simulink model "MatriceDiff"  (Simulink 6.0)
settings: Solver=ode45  StartTime=0  StopTime=17*t0  RelTol=1e-3
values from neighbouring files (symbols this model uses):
  b = S/Sm    (= 0.1)    [Constantes.m]    (also in ConstantesBck.m)
  beta = 0.95    [Constantes.m]    (also in ConstantesBck.m; ResCourV1.m = 1; ResCrV1.m = 1; ResEnerV1.m = 1)
  C = 1    [Constantes.m]    (also in ConstantesBck.m)
  gk = 36    [Constantes.m]    (also in ConstantesBck.m; sim_hh.m)
  gl = 0.3    [Constantes.m]    (also in ConstantesBck.m; sim_hh.m)
  gna = 120    [Constantes.m]    (also in ConstantesBck.m; sim_hh.m)
  h0 = 0.5961    [Constantes.m]    (also in ConstantesBck.m)
  m0 = 0.0529    [Constantes.m]    (also in ConstantesBck.m)
  mK = 0    [Constantes.m]    (also in ConstantesBck.m)
  mL = 0    [Constantes.m]    (also in ConstantesBck.m)
  mNa = 0    [Constantes.m]    (also in ConstantesBck.m)
  N = [6,8,5,5,7,1,2,6,9,1,1,9,4,8,8,7]    [Constantes.m]    (also in ConstantesBck.m; ImpedanceZtissus.m = 100; Ztissus.m = 100; charge.m = N(:,2))
  n0 = 0.3177    [Constantes.m]    (also in ConstantesBck.m)
  rapportIE = 10    [Constantes.m]
  Sm = 3.14e-2    (= 0.0314)    [Constantes.m]    (also in ConstantesBck.m = 0.000314)
  t0 = 2E-3    (= 0.002)    [Constantes.m]    (also in ConstantesBck.m = 0.001)
  Vk = -82    [Constantes.m]    (also in ConstantesBck.m)
  Vl = -59    [Constantes.m]    (also in ConstantesBck.m)
  Vna = 45    [Constantes.m]    (also in ConstantesBck.m)
  Vr = -70    [Constantes.m]    (also in ConstantesBck.m)
undefined symbols (not defined in the file or in its folder): ln
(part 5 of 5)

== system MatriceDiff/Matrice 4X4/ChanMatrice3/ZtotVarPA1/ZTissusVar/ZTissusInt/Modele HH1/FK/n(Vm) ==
  note: V
  note: alpha_*(1-n)
  note: beta_n*n
  note: n
  note: n
  Vm : Inport  Port=1  LatchInput=off
  (1-n) : Fcn  Expr=1-u
  Integrator1 : Integrator  InitialCondition=n0
  Product : Product
  Product1 : Product
  Sum1 : Sum  Inputs=+-
  V : Fcn  Expr=u-Vr
  alpha_n : Fcn  Expr=(0.01*(10-u))/(exp((10-u)/10)-1)
  beta_n : Fcn  Expr=0.125*exp(-u/80)
  n : Outport  InitialOutput=0
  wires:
  V/1 -> alpha_n/1, beta_n/1
  alpha_n/1 -> Product/2
  (1-n)/1 -> Product/1
  beta_n/1 -> Product1/1
  Product/1 -> Sum1/1
  Product1/1 -> Sum1/2
  Sum1/1 -> Integrator1/1
  Integrator1/1 -> (1-n)/1, Product1/2, n/1
  Vm/1 -> V/1

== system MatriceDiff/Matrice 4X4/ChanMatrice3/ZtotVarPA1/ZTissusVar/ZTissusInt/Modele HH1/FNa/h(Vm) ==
  note: h
  note: h
  note: beta_h*h
  note: alpha_h*(1-h)
  note: V
  Vm : Inport  Port=1  LatchInput=off
  (1-h) : Fcn  Expr=1-u
  Integrator1 : Integrator  InitialCondition=h0
  Product : Product
  Product1 : Product
  Sum1 : Sum  Inputs=+-
  V : Fcn  Expr=u-Vr
  alpha_h : Fcn  Expr=0.07*exp(-u/20)
  beta_h : Fcn  Expr=1/(exp((30-u)/10)+1)
  h : Outport  InitialOutput=0
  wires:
  Vm/1 -> V/1
  Integrator1/1 -> h/1, Product1/2, (1-h)/1
  Sum1/1 -> Integrator1/1
  Product1/1 -> Sum1/2
  Product/1 -> Sum1/1
  beta_h/1 -> Product1/1
  (1-h)/1 -> Product/1
  alpha_h/1 -> Product/2
  V/1 -> beta_h/1, alpha_h/1

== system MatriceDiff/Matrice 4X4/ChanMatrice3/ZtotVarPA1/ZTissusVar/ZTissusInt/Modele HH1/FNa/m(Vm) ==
  note: m
  note: m
  note: beta_m*m
  note: alpha_m*(1-m)
  note: V
  Vm : Inport  Port=1  LatchInput=off
  (1-m) : Fcn  Expr=1-u
  Integrator1 : Integrator  InitialCondition=m0
  Product : Product
  Product1 : Product
  Sum1 : Sum  Inputs=+-
  V : Fcn  Expr=u-Vr
  alpha_m : Fcn  Expr=(0.1*(25-u))/(exp((25-u)/10)-1)
  beta_m : Fcn  Expr=4*exp(-u/18)
  n : Outport  InitialOutput=0
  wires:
  Vm/1 -> V/1
  Integrator1/1 -> n/1, Product1/2, (1-m)/1
  Sum1/1 -> Integrator1/1
  Product1/1 -> Sum1/2
  Product/1 -> Sum1/1
  beta_m/1 -> Product1/1
  (1-m)/1 -> Product/1
  alpha_m/1 -> Product/2
  V/1 -> beta_m/1, alpha_m/1

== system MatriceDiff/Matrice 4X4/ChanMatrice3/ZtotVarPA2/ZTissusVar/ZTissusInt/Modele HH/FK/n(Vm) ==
  note: V
  note: alpha_*(1-n)
  note: beta_n*n
  note: n
  note: n
  Vm : Inport  Port=1  LatchInput=off
  (1-n) : Fcn  Expr=1-u
  Integrator1 : Integrator  InitialCondition=n0
  Product : Product
  Product1 : Product
  Sum1 : Sum  Inputs=+-
  V : Fcn  Expr=u-Vr
  alpha_n : Fcn  Expr=(0.01*(10-u))/(exp((10-u)/10)-1)
  beta_n : Fcn  Expr=0.125*exp(-u/80)
  n : Outport  InitialOutput=0
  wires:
  V/1 -> alpha_n/1, beta_n/1
  alpha_n/1 -> Product/2
  (1-n)/1 -> Product/1
  beta_n/1 -> Product1/1
  Product/1 -> Sum1/1
  Product1/1 -> Sum1/2
  Sum1/1 -> Integrator1/1
  Integrator1/1 -> (1-n)/1, Product1/2, n/1
  Vm/1 -> V/1

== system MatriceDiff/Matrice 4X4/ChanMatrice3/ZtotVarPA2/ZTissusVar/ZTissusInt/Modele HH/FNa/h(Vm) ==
  note: h
  note: h
  note: beta_h*h
  note: alpha_h*(1-h)
  note: V
  Vm : Inport  Port=1  LatchInput=off
  (1-h) : Fcn  Expr=1-u
  Integrator1 : Integrator  InitialCondition=h0
  Product : Product
  Product1 : Product
  Sum1 : Sum  Inputs=+-
  V : Fcn  Expr=u-Vr
  alpha_h : Fcn  Expr=0.07*exp(-u/20)
  beta_h : Fcn  Expr=1/(exp((30-u)/10)+1)
  h : Outport  InitialOutput=0
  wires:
  Vm/1 -> V/1
  Integrator1/1 -> h/1, Product1/2, (1-h)/1
  Sum1/1 -> Integrator1/1
  Product1/1 -> Sum1/2
  Product/1 -> Sum1/1
  beta_h/1 -> Product1/1
  (1-h)/1 -> Product/1
  alpha_h/1 -> Product/2
  V/1 -> beta_h/1, alpha_h/1

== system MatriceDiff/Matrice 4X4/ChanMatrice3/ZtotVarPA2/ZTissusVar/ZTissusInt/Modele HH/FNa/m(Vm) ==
  note: m
  note: m
  note: beta_m*m
  note: alpha_m*(1-m)
  note: V
  Vm : Inport  Port=1  LatchInput=off
  (1-m) : Fcn  Expr=1-u
  Integrator1 : Integrator  InitialCondition=m0
  Product : Product
  Product1 : Product
  Sum1 : Sum  Inputs=+-
  V : Fcn  Expr=u-Vr
  alpha_m : Fcn  Expr=(0.1*(25-u))/(exp((25-u)/10)-1)
  beta_m : Fcn  Expr=4*exp(-u/18)
  n : Outport  InitialOutput=0
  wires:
  Vm/1 -> V/1
  Integrator1/1 -> n/1, Product1/2, (1-m)/1
  Sum1/1 -> Integrator1/1
  Product1/1 -> Sum1/2
  Product/1 -> Sum1/1
  beta_m/1 -> Product1/1
  (1-m)/1 -> Product/1
  alpha_m/1 -> Product/2
  V/1 -> beta_m/1, alpha_m/1

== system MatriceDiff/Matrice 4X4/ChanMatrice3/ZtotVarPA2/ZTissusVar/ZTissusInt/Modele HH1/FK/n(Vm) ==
  note: V
  note: alpha_*(1-n)
  note: beta_n*n
  note: n
  note: n
  Vm : Inport  Port=1  LatchInput=off
  (1-n) : Fcn  Expr=1-u
  Integrator1 : Integrator  InitialCondition=n0
  Product : Product
  Product1 : Product
  Sum1 : Sum  Inputs=+-
  V : Fcn  Expr=u-Vr
  alpha_n : Fcn  Expr=(0.01*(10-u))/(exp((10-u)/10)-1)
  beta_n : Fcn  Expr=0.125*exp(-u/80)
  n : Outport  InitialOutput=0
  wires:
  V/1 -> alpha_n/1, beta_n/1
  alpha_n/1 -> Product/2
  (1-n)/1 -> Product/1
  beta_n/1 -> Product1/1
  Product/1 -> Sum1/1
  Product1/1 -> Sum1/2
  Sum1/1 -> Integrator1/1
  Integrator1/1 -> (1-n)/1, Product1/2, n/1
  Vm/1 -> V/1

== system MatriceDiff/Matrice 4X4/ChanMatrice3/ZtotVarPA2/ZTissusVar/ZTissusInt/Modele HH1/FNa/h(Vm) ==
  note: h
  note: h
  note: beta_h*h
  note: alpha_h*(1-h)
  note: V
  Vm : Inport  Port=1  LatchInput=off
  (1-h) : Fcn  Expr=1-u
  Integrator1 : Integrator  InitialCondition=h0
  Product : Product
  Product1 : Product
  Sum1 : Sum  Inputs=+-
  V : Fcn  Expr=u-Vr
  alpha_h : Fcn  Expr=0.07*exp(-u/20)
  beta_h : Fcn  Expr=1/(exp((30-u)/10)+1)
  h : Outport  InitialOutput=0
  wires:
  Vm/1 -> V/1
  Integrator1/1 -> h/1, Product1/2, (1-h)/1
  Sum1/1 -> Integrator1/1
  Product1/1 -> Sum1/2
  Product/1 -> Sum1/1
  beta_h/1 -> Product1/1
  (1-h)/1 -> Product/1
  alpha_h/1 -> Product/2
  V/1 -> beta_h/1, alpha_h/1

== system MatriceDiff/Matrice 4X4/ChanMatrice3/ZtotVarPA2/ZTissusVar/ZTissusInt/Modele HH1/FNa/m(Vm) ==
  note: m
  note: m
  note: beta_m*m
  note: alpha_m*(1-m)
  note: V
  Vm : Inport  Port=1  LatchInput=off
  (1-m) : Fcn  Expr=1-u
  Integrator1 : Integrator  InitialCondition=m0
  Product : Product
  Product1 : Product
  Sum1 : Sum  Inputs=+-
  V : Fcn  Expr=u-Vr
  alpha_m : Fcn  Expr=(0.1*(25-u))/(exp((25-u)/10)-1)
  beta_m : Fcn  Expr=4*exp(-u/18)
  n : Outport  InitialOutput=0
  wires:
  Vm/1 -> V/1
  Integrator1/1 -> n/1, Product1/2, (1-m)/1
  Sum1/1 -> Integrator1/1
  Product1/1 -> Sum1/2
  Product/1 -> Sum1/1
  beta_m/1 -> Product1/1
  (1-m)/1 -> Product/1
  alpha_m/1 -> Product/2
  V/1 -> beta_m/1, alpha_m/1

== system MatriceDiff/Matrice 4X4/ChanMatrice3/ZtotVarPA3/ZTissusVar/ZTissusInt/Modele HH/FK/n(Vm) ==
  note: V
  note: alpha_*(1-n)
  note: beta_n*n
  note: n
  note: n
  Vm : Inport  Port=1  LatchInput=off
  (1-n) : Fcn  Expr=1-u
  Integrator1 : Integrator  InitialCondition=n0
  Product : Product
  Product1 : Product
  Sum1 : Sum  Inputs=+-
  V : Fcn  Expr=u-Vr
  alpha_n : Fcn  Expr=(0.01*(10-u))/(exp((10-u)/10)-1)
  beta_n : Fcn  Expr=0.125*exp(-u/80)
  n : Outport  InitialOutput=0
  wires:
  V/1 -> alpha_n/1, beta_n/1
  alpha_n/1 -> Product/2
  (1-n)/1 -> Product/1
  beta_n/1 -> Product1/1
  Product/1 -> Sum1/1
  Product1/1 -> Sum1/2
  Sum1/1 -> Integrator1/1
  Integrator1/1 -> (1-n)/1, Product1/2, n/1
  Vm/1 -> V/1

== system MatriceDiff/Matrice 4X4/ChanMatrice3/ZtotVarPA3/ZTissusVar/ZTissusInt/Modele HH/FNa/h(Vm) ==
  note: h
  note: h
  note: beta_h*h
  note: alpha_h*(1-h)
  note: V
  Vm : Inport  Port=1  LatchInput=off
  (1-h) : Fcn  Expr=1-u
  Integrator1 : Integrator  InitialCondition=h0
  Product : Product
  Product1 : Product
  Sum1 : Sum  Inputs=+-
  V : Fcn  Expr=u-Vr
  alpha_h : Fcn  Expr=0.07*exp(-u/20)
  beta_h : Fcn  Expr=1/(exp((30-u)/10)+1)
  h : Outport  InitialOutput=0
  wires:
  Vm/1 -> V/1
  Integrator1/1 -> h/1, Product1/2, (1-h)/1
  Sum1/1 -> Integrator1/1
  Product1/1 -> Sum1/2
  Product/1 -> Sum1/1
  beta_h/1 -> Product1/1
  (1-h)/1 -> Product/1
  alpha_h/1 -> Product/2
  V/1 -> beta_h/1, alpha_h/1

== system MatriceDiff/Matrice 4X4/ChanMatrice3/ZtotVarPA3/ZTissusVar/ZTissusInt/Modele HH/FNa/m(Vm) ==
  note: m
  note: m
  note: beta_m*m
  note: alpha_m*(1-m)
  note: V
  Vm : Inport  Port=1  LatchInput=off
  (1-m) : Fcn  Expr=1-u
  Integrator1 : Integrator  InitialCondition=m0
  Product : Product
  Product1 : Product
  Sum1 : Sum  Inputs=+-
  V : Fcn  Expr=u-Vr
  alpha_m : Fcn  Expr=(0.1*(25-u))/(exp((25-u)/10)-1)
  beta_m : Fcn  Expr=4*exp(-u/18)
  n : Outport  InitialOutput=0
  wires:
  Vm/1 -> V/1
  Integrator1/1 -> n/1, Product1/2, (1-m)/1
  Sum1/1 -> Integrator1/1
  Product1/1 -> Sum1/2
  Product/1 -> Sum1/1
  beta_m/1 -> Product1/1
  (1-m)/1 -> Product/1
  alpha_m/1 -> Product/2
  V/1 -> beta_m/1, alpha_m/1

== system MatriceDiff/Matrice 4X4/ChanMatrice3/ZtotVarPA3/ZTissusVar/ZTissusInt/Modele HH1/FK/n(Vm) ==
  note: V
  note: alpha_*(1-n)
  note: beta_n*n
  note: n
  note: n
  Vm : Inport  Port=1  LatchInput=off
  (1-n) : Fcn  Expr=1-u
  Integrator1 : Integrator  InitialCondition=n0
  Product : Product
  Product1 : Product
  Sum1 : Sum  Inputs=+-
  V : Fcn  Expr=u-Vr
  alpha_n : Fcn  Expr=(0.01*(10-u))/(exp((10-u)/10)-1)
  beta_n : Fcn  Expr=0.125*exp(-u/80)
  n : Outport  InitialOutput=0
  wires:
  V/1 -> alpha_n/1, beta_n/1
  alpha_n/1 -> Product/2
  (1-n)/1 -> Product/1
  beta_n/1 -> Product1/1
  Product/1 -> Sum1/1
  Product1/1 -> Sum1/2
  Sum1/1 -> Integrator1/1
  Integrator1/1 -> (1-n)/1, Product1/2, n/1
  Vm/1 -> V/1

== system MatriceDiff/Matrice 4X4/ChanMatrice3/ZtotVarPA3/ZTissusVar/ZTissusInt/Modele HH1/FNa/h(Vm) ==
  note: h
  note: h
  note: beta_h*h
  note: alpha_h*(1-h)
  note: V
  Vm : Inport  Port=1  LatchInput=off
  (1-h) : Fcn  Expr=1-u
  Integrator1 : Integrator  InitialCondition=h0
  Product : Product
  Product1 : Product
  Sum1 : Sum  Inputs=+-
  V : Fcn  Expr=u-Vr
  alpha_h : Fcn  Expr=0.07*exp(-u/20)
  beta_h : Fcn  Expr=1/(exp((30-u)/10)+1)
  h : Outport  InitialOutput=0
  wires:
  Vm/1 -> V/1
  Integrator1/1 -> h/1, Product1/2, (1-h)/1
  Sum1/1 -> Integrator1/1
  Product1/1 -> Sum1/2
  Product/1 -> Sum1/1
  beta_h/1 -> Product1/1
  (1-h)/1 -> Product/1
  alpha_h/1 -> Product/2
  V/1 -> beta_h/1, alpha_h/1

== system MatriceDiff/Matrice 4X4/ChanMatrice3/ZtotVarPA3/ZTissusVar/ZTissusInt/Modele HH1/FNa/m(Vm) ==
  note: m
  note: m
  note: beta_m*m
  note: alpha_m*(1-m)
  note: V
  Vm : Inport  Port=1  LatchInput=off
  (1-m) : Fcn  Expr=1-u
  Integrator1 : Integrator  InitialCondition=m0
  Product : Product
  Product1 : Product
  Sum1 : Sum  Inputs=+-
  V : Fcn  Expr=u-Vr
  alpha_m : Fcn  Expr=(0.1*(25-u))/(exp((25-u)/10)-1)
  beta_m : Fcn  Expr=4*exp(-u/18)
  n : Outport  InitialOutput=0
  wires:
  Vm/1 -> V/1
  Integrator1/1 -> n/1, Product1/2, (1-m)/1
  Sum1/1 -> Integrator1/1
  Product1/1 -> Sum1/2
  Product/1 -> Sum1/1
  beta_m/1 -> Product1/1
  (1-m)/1 -> Product/1
  alpha_m/1 -> Product/2
  V/1 -> beta_m/1, alpha_m/1

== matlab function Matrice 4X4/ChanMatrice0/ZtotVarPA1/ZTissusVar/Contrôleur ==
function [y,temp] = fcn(u,calc)
% This block supports an embeddable subset of the MATLAB language.
% See the help menu for details. 

if u == 0
    y = 0;
    temp = 1E-6;
else
    y = calc;
    temp = u;
end

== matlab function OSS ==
function [S0,Ref0,S1,Ref1,S2,Ref2,S3,Ref3,S4,Ref4,S5,Ref5,S6,Ref6,S7,Ref7,S8,Ref8,S9,Ref9,S10,Ref10,S11,Ref11,S12,Ref12,S13,Ref13,S14,Ref14,S15,Ref15,MatCourant] = fcn(u0,u1,u2,u3,u4,u5,u6,u7,u8,u9,u10,u11,u12,u13,u14,u15,tc0,tc1,tc2,dyn,rst)
%Fonction qui détermine les endroits à stimuler pour obtenir une puissance 
%moyenne par canal minimal

%Valeur utilisée
Vdd=3.3*3.14e-2*(1-0.1)*1000; %mV
Imax=200E-6;

%Enregistrement de l'indice et de l'amplitude pour chaque canal
IndAmpChan0=[1,2,3,4;u0,u1,u2,u3];
IndAmpChan1=[5,6,7,8;u4,u5,u6,u7];
IndAmpChan2=[9,10,11,12;u8,u9,u10,u11];
IndAmpChan3=[13,14,15,16;u12,u13,u14,u15];

%Premier tri
for k=1:2
    for i=1:3
        if(IndAmpChan0(2,i)>IndAmpChan0(2,i+1))
            temp=IndAmpChan0(:,i+1);
            IndAmpChan0(:,i+1)=IndAmpChan0(:,i);
            IndAmpChan0(:,i)=temp;        
        end
        if(IndAmpChan1(2,i)<IndAmpChan1(2,i+1))
            temp=IndAmpChan1(:,i+1);
            IndAmpChan1(:,i+1)=IndAmpChan1(:,i);
            IndAmpChan1(:,i)=temp;        
        end    
        if(IndAmpChan2(2,i)>IndAmpChan2(2,i+1))
            temp=IndAmpChan2(:,i+1);
            IndAmpChan2(:,i+1)=IndAmpChan2(:,i);
            IndAmpChan2(:,i)=temp;        
        end    
        if(IndAmpChan3(2,i)<IndAmpChan3(2,i+1))
            temp=IndAmpChan3(:,i+1);
            IndAmpChan3(:,i+1)=IndAmpChan3(:,i);
            IndAmpChan3(:,i)=temp;        
        end        
    end
end

%On regroupe les lignes 2 par deux
sump1=[0,0,0,0];
sump2=[0,0,0,0];
for i=1:4
    sump1(i)=IndAmpChan0(2,i)+IndAmpChan1(2,i);
    sump2(i)=IndAmpChan2(2,i)+IndAmpChan3(2,i);
end

%2e tri
for k=1:2
    for i=1:3
        if(sump1(i)>sump1(i+1))
            temp=IndAmpChan0(:,i+1);
            IndAmpChan0(:,i+1)=IndAmpChan0(:,i);
            IndAmpChan0(:,i)=temp; 
            
            temp=IndAmpChan1(:,i+1);
            IndAmpChan1(:,i+1)=IndAmpChan1(:,i);
            IndAmpChan1(:,i)=temp;
            
            tempo=sump1(i+1);
            sump1(i+1)=sump1(i);
            sump1(i)=tempo;            
        end  
        if(sump2(i)<sump2(i+1))
            temp=IndAmpChan2(:,i+1);
            IndAmpChan2(:,i+1)=IndAmpChan2(:,i);
            IndAmpChan2(:,i)=temp;        
            
            temp=IndAmpChan3(:,i+1);
            IndAmpChan3(:,i+1)=IndAmpChan3(:,i);
            IndAmpChan3(:,i)=temp;        
            
            tempo=sump2(i+1);
            sump2(i+1)=sump2(i);
            sump2(i)=tempo;             
        end   
    end
end

if(tc0==0)
    Signe=-1;
else
    Signe=1;
end

%Initialisation des tableaux de sorties
SOut=[0,0,0,0,0,0,0,0,0,0,0,0,0,0,0,0];

%Détermination des sorties actives
if(tc2 == 0)
    if(tc1 == 0)
        i=1;
    else
        i=2;
    end
else
    if(tc1 == 0)
        i=3;
    else
        i=4;
    end    
end

RefOut=0;
if not(rst == 0)
    %Calcul des valeurs à sortir
    %La référence se doit d'être la même puisqu'il ne s'agit que d'une seule électrode
    SOut(IndAmpChan0(1,i))=Signe*Imax*IndAmpChan0(2,i)/10;
    SOut(IndAmpChan1(1,i))=Signe*Imax*IndAmpChan1(2,i)/10;
    SOut(IndAmpChan2(1,i))=Signe*Imax*IndAmpChan2(2,i)/10;
    SOut(IndAmpChan3(1,i))=Signe*Imax*IndAmpChan3(2,i)/10;

    RefOut=-1*Signe*Vdd*dyn;
end

%Assignation des sorties
S0=SOut(1);
Ref0=RefOut;
S1=SOut(2);
Ref1=RefOut;
S2=SOut(3);
Ref2=RefOut;
S3=SOut(4);
Ref3=RefOut;
S4=SOut(5);
Ref4=RefOut;
S5=SOut(6);
Ref5=RefOut;
S6=SOut(7);
Ref6=RefOut;
S7=SOut(8);
Ref7=RefOut;
S8=SOut(9);
Ref8=RefOut;
S9=SOut(10);
Ref9=RefOut;
S10=SOut(11);
Ref10=RefOut;
S11=SOut(12);
Ref11=RefOut;
S12=SOut(13);
Ref12=RefOut;
S13=SOut(14);
Ref13=RefOut;
S14=SOut(15);
Ref14=RefOut;
S15=SOut(16);
Ref15=RefOut;
MatCourant=SOut;

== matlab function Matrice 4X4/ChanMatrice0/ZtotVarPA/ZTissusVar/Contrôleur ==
function [y,temp] = fcn(u,calc)
% This block supports an embeddable subset of the MATLAB language.
% See the help menu for details. 

if u == 0
    y = 0;
    temp = 1E-6;
else
    y = calc;
    temp = u;
end

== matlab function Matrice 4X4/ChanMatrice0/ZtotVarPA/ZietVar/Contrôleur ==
function [y,temp] = fcn(u,calc)
% This block supports an embeddable subset of the MATLAB language.
% See the help menu for details. 

if u == 0
    y = 0;
    temp = 1E-6;
else
    y = calc;
    temp = u;
end

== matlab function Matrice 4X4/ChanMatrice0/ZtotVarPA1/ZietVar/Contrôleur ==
function [y,temp] = fcn(u,calc)
% This block supports an embeddable subset of the MATLAB language.
% See the help menu for details. 

if u == 0
    y = 0;
    temp = 1E-6;
else
    y = calc;
    temp = u;
end

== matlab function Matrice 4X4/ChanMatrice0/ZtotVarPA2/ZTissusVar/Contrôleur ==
function [y,temp] = fcn(u,calc)
% This block supports an embeddable subset of the MATLAB language.
% See the help menu for details. 

if u == 0
    y = 0;
    temp = 1E-6;
else
    y = calc;
    temp = u;
end

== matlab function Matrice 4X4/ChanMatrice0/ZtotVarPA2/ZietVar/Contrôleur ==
function [y,temp] = fcn(u,calc)
% This block supports an embeddable subset of the MATLAB language.
% See the help menu for details. 

if u == 0
    y = 0;
    temp = 1E-6;
else
    y = calc;
    temp = u;
end

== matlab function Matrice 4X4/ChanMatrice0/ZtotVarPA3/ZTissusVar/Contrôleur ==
function [y,temp] = fcn(u,calc)
% This block supports an embeddable subset of the MATLAB language.
% See the help menu for details. 

if u == 0
    y = 0;
    temp = 1E-6;
else
    y = calc;
    temp = u;
end

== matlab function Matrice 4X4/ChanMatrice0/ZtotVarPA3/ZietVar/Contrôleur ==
function [y,temp] = fcn(u,calc)
% This block supports an embeddable subset of the MATLAB language.
% See the help menu for details. 

if u == 0
    y = 0;
    temp = 1E-6;
else
    y = calc;
    temp = u;
end

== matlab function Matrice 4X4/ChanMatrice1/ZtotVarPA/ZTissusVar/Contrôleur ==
function [y,temp] = fcn(u,calc)
% This block supports an embeddable subset of the MATLAB language.
% See the help menu for details. 

if u == 0
    y = 0;
    temp = 1E-6;
else
    y = calc;
    temp = u;
end

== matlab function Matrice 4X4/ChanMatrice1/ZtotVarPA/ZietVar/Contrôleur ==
function [y,temp] = fcn(u,calc)
% This block supports an embeddable subset of the MATLAB language.
% See the help menu for details. 

if u == 0
    y = 0;
    temp = 1E-6;
else
    y = calc;
    temp = u;
end

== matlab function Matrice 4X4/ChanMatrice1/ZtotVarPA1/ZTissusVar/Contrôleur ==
function [y,temp] = fcn(u,calc)
% This block supports an embeddable subset of the MATLAB language.
% See the help menu for details. 

if u == 0
    y = 0;
    temp = 1E-6;
else
    y = calc;
    temp = u;
end

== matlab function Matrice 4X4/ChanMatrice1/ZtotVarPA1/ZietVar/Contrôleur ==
function [y,temp] = fcn(u,calc)
% This block supports an embeddable subset of the MATLAB language.
% See the help menu for details. 

if u == 0
    y = 0;
    temp = 1E-6;
else
    y = calc;
    temp = u;
end

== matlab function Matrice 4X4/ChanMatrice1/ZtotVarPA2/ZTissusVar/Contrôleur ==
function [y,temp] = fcn(u,calc)
% This block supports an embeddable subset of the MATLAB language.
% See the help menu for details. 

if u == 0
    y = 0;
    temp = 1E-6;
else
    y = calc;
    temp = u;
end

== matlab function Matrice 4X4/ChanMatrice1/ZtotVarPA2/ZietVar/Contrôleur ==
function [y,temp] = fcn(u,calc)
% This block supports an embeddable subset of the MATLAB language.
% See the help menu for details. 

if u == 0
    y = 0;
    temp = 1E-6;
else
    y = calc;
    temp = u;
end

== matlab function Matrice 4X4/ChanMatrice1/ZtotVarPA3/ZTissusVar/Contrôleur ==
function [y,temp] = fcn(u,calc)
% This block supports an embeddable subset of the MATLAB language.
% See the help menu for details. 

if u == 0
    y = 0;
    temp = 1E-6;
else
    y = calc;
    temp = u;
end

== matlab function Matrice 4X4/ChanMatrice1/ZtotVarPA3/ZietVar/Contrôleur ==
function [y,temp] = fcn(u,calc)
% This block supports an embeddable subset of the MATLAB language.
% See the help menu for details. 

if u == 0
    y = 0;
    temp = 1E-6;
else
    y = calc;
    temp = u;
end

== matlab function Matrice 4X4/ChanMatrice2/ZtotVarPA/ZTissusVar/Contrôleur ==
function [y,temp] = fcn(u,calc)
% This block supports an embeddable subset of the MATLAB language.
% See the help menu for details. 

if u == 0
    y = 0;
    temp = 1E-6;
else
    y = calc;
    temp = u;
end

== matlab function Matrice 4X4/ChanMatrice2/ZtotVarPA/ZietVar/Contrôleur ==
function [y,temp] = fcn(u,calc)
% This block supports an embeddable subset of the MATLAB language.
% See the help menu for details. 

if u == 0
    y = 0;
    temp = 1E-6;
else
    y = calc;
    temp = u;
end

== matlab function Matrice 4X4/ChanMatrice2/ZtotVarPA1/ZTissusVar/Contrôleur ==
function [y,temp] = fcn(u,calc)
% This block supports an embeddable subset of the MATLAB language.
% See the help menu for details. 

if u == 0
    y = 0;
    temp = 1E-6;
else
    y = calc;
    temp = u;
end

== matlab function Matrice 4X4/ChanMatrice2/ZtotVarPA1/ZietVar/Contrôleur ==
function [y,temp] = fcn(u,calc)
% This block supports an embeddable subset of the MATLAB language.
% See the help menu for details. 

if u == 0
    y = 0;
    temp = 1E-6;
else
    y = calc;
    temp = u;
end

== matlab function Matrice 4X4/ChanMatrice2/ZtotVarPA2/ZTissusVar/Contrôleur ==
function [y,temp] = fcn(u,calc)
% This block supports an embeddable subset of the MATLAB language.
% See the help menu for details. 

if u == 0
    y = 0;
    temp = 1E-6;
else
    y = calc;
    temp = u;
end

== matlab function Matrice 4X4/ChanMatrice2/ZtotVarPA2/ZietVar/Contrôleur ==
function [y,temp] = fcn(u,calc)
% This block supports an embeddable subset of the MATLAB language.
% See the help menu for details. 

if u == 0
    y = 0;
    temp = 1E-6;
else
    y = calc;
    temp = u;
end

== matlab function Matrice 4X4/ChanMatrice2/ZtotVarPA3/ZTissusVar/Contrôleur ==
function [y,temp] = fcn(u,calc)
% This block supports an embeddable subset of the MATLAB language.
% See the help menu for details. 

if u == 0
    y = 0;
    temp = 1E-6;
else
    y = calc;
    temp = u;
end

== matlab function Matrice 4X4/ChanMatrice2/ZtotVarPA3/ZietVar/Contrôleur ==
function [y,temp] = fcn(u,calc)
% This block supports an embeddable subset of the MATLAB language.
% See the help menu for details. 

if u == 0
    y = 0;
    temp = 1E-6;
else
    y = calc;
    temp = u;
end

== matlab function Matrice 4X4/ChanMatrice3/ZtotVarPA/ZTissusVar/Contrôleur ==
function [y,temp] = fcn(u,calc)
% This block supports an embeddable subset of the MATLAB language.
% See the help menu for details. 

if u == 0
    y = 0;
    temp = 1E-6;
else
    y = calc;
    temp = u;
end

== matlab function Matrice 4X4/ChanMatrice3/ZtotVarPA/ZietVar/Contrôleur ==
function [y,temp] = fcn(u,calc)
% This block supports an embeddable subset of the MATLAB language.
% See the help menu for details. 

if u == 0
    y = 0;
    temp = 1E-6;
else
    y = calc;
    temp = u;
end

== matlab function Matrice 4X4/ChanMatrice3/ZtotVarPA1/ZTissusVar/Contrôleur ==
function [y,temp] = fcn(u,calc)
% This block supports an embeddable subset of the MATLAB language.
% See the help menu for details. 

if u == 0
    y = 0;
    temp = 1E-6;
else
    y = calc;
    temp = u;
end

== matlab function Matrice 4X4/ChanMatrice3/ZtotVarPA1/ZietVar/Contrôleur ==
function [y,temp] = fcn(u,calc)
% This block supports an embeddable subset of the MATLAB language.
% See the help menu for details. 

if u == 0
    y = 0;
    temp = 1E-6;
else
    y = calc;
    temp = u;
end

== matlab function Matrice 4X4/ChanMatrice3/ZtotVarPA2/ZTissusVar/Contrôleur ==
function [y,temp] = fcn(u,calc)
% This block supports an embeddable subset of the MATLAB language.
% See the help menu for details. 

if u == 0
    y = 0;
    temp = 1E-6;
else
    y = calc;
    temp = u;
end

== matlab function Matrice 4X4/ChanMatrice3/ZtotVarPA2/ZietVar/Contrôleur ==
function [y,temp] = fcn(u,calc)
% This block supports an embeddable subset of the MATLAB language.
% See the help menu for details. 

if u == 0
    y = 0;
    temp = 1E-6;
else
    y = calc;
    temp = u;
end

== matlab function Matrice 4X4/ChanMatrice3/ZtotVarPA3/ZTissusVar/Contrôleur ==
function [y,temp] = fcn(u,calc)
% This block supports an embeddable subset of the MATLAB language.
% See the help menu for details. 

if u == 0
    y = 0;
    temp = 1E-6;
else
    y = calc;
    temp = u;
end

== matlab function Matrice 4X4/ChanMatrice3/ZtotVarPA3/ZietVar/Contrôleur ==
function [y,temp] = fcn(u,calc)
% This block supports an embeddable subset of the MATLAB language.
% See the help menu for details. 

if u == 0
    y = 0;
    temp = 1E-6;
else
    y = calc;
    temp = u;
end
